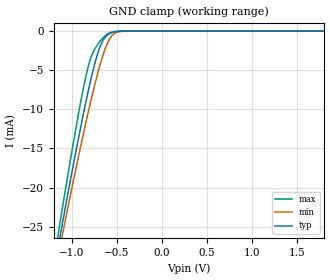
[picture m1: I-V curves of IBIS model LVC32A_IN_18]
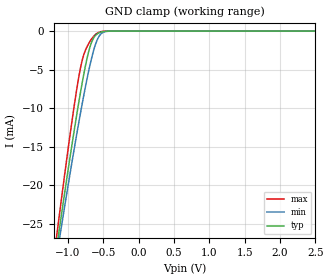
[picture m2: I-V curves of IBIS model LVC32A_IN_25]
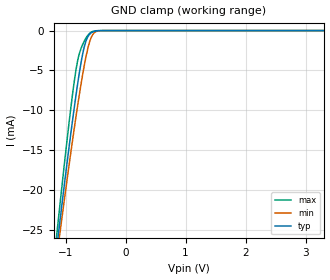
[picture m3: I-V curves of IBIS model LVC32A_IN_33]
| TEXAS INSTRUMENTS INCORPORATED
| Standard Linear and Logic Group
| IBIS Model of SN74LVC32A
| QUADRUPLE 2-INPUT POSITIVE-OR GATES
| This file contains package information for the following:
|  SOIC 14-pin (D) package as [Component] LVC32A_D
|  SOP  14-pin (NS) package as [Component] LVC32A_NS
|  SSOP 14-pin (DB) package as [Component] LVC32A_DB
|  TSSOP 14-pin (PW) package as [Component] LVC32A_PW
|  QFN 14-pin (RGY) package as [Componenet] LVC32A_RGY
| This device can be powered at the following Vccs:
|  1.8 volt Vcc
|  2.5 volt Vcc
|  3.3 volt Vcc
| This file provides unique models under the [Model Selector] for each Vcc.
| For operation at a specific Vcc, select the appropriate model after each
| [Model Selector] keyword.
[IBIS Ver]   3.2
[Comment char]  |_char
[File Name]   sn74lvc32a.ibs
[File Rev]   1.2 | k_die
[Date]   August 19, 2003
[Source]   Data created from TI-SPICE simulations at TI-SLL.
[Notes]   The following is an IBIS list for the LVC32A.
   Please contact sllibis@ti.com with questions and
   comments concerning SLL IBIS models.
   - Power clamp data deleted as there is no power-clamp diode.
[Disclaimer] Property of Texas Instruments Incorporated.  Unauthorized
   reproduction and/or distribution is strictly prohibited.
   This product is protected under copyright law.
   Created  2002, (C) Copyright  2002, Texas Instruments
   Incorporated, All Rights Reserved
   UNLESS THERE IS A SIGNED, WRITTEN AGREEMENT TO THE
   CONTRARY, TEXAS INSTRUMENTS (TI) IS PROVIDING THE IBIS
   MODELS  AND WITHOUT ANY WARRANTY, EXPRESSED OR
   IMPLIED.  TI assumes no liability for:
   1) the accuracy of the IBIS models provided to your
   company;
   2) the proper functioning of these IBIS Models in your
   design or for any resulting applications; or
   3) infringement of patents, copyrights or intellectual
   property rights resulting from your use of these IBIS
   models.
   TI provides IBIS Models as a service to our customers.
   You and your company shall not distribute, sell or give
   these models to anyone else without prior written
   permission from TI.
   TI reserves the right to make changes to our products or
   to discontinue any semiconductor product or service
   without notice, and advises our customers to obtain the
   latest version of relevant information to verify, before
   placing orders, that the information being relied on is
   current.
   Please be aware that your receipt and use of the IBIS
   information provided shall serve as acceptance of these
   terms and conditions.  If you do not accept these terms,
   you should return or destroy the IBIS models and any
   other accompanying information immediately.
| Component LVC32A_D 14-pin SOIC
[Component]   LVC32A_D
[Manufacturer]   Texas Instruments, Inc.
[Package]
|   typ   min   max
R_pkg   3.100e-02   2.800e-02   3.400e-02
L_pkg   3.109e-09   2.462e-09   3.889e-09
C_pkg   4.730e-13   3.630e-13   6.280e-13
[Pin]   signal_name   model_name   R_pin   L_pin   C_pin
1   1A   LVC32A_IN   3.300e-02   3.854e-09   6.220e-13
2   1B   LVC32A_IN   3.200e-02   3.188e-09   4.730e-13
3   1Y   LVC32A_OUT   2.800e-02   2.462e-09   3.770e-13
4   2A   LVC32A_IN   3.100e-02   2.596e-09   3.630e-13
5   2B   LVC32A_IN   2.800e-02   2.521e-09   3.720e-13
6   2Y   LVC32A_OUT   3.400e-02   3.250e-09   4.760e-13
7   GND   GND   3.400e-02   3.889e-09   6.280e-13
8   3Y   LVC32A_OUT   3.400e-02   3.889e-09   6.280e-13
9   3A   LVC32A_IN   3.400e-02   3.250e-09   4.760e-13
10   3B   LVC32A_IN   2.800e-02   2.521e-09   3.720e-13
11   4Y   LVC32A_OUT   3.100e-02   2.596e-09   3.640e-13
12   4A   LVC32A_IN   2.800e-02   2.462e-09   3.770e-13
13   4B   LVC32A_IN   3.200e-02   3.188e-09   4.730e-13
14   VCC   POWER   3.300e-02   3.854e-09   6.220e-13
| Component LVC32A_DB 14-pin SSOP
[Component]   LVC32A_DB
[Manufacturer]   Texas Instruments, Inc.
[Package]
|   typ   min   max
R_pkg   4.400e-02   4.100e-02   4.600e-02
L_pkg   3.551e-09   3.258e-09   3.927e-09
C_pkg   4.020e-13   3.600e-13   4.210e-13
[Pin]   signal_name   model_name   R_pin   L_pin   C_pin
1   1A   LVC32A_IN   4.600e-02   3.927e-09   4.080e-13
2   1B   LVC32A_IN   4.400e-02   3.587e-09   4.210e-13
3   1Y   LVC32A_OUT   4.100e-02   3.289e-09   3.980e-13
4   2A   LVC32A_IN   4.200e-02   3.258e-09   3.600e-13
5   2B   LVC32A_IN   4.100e-02   3.286e-09   4.030e-13
6   2Y   LVC32A_OUT   4.400e-02   3.586e-09   4.210e-13
7   GND   GND   4.600e-02   3.927e-09   4.080e-13
8   3Y   LVC32A_OUT   4.600e-02   3.927e-09   4.080e-13
9   3A   LVC32A_IN   4.400e-02   3.586e-09   4.210e-13
10   3B   LVC32A_IN   4.100e-02   3.286e-09   4.030e-13
11   4Y   LVC32A_OUT   4.300e-02   3.258e-09   3.600e-13
12   4A   LVC32A_IN   4.100e-02   3.289e-09   3.980e-13
13   4B   LVC32A_IN   4.400e-02   3.587e-09   4.210e-13
14   VCC   POWER   4.600e-02   3.927e-09   4.080e-13
| Component LVC126A_NS 14-pin SOP
[Component]   LVC32A_NS
[Manufacturer]  Texas Instruments, Inc.
[Package]
|   typ   min   max
R_pkg   4.500e-02   3.900e-02   5.400e-02
L_pkg   3.796e-09   2.561e-09   4.952e-09
C_pkg   5.280e-13   2.880e-13   7.100e-13
[Pin]   signal_name   model_name   R_pin   L_pin   C_pin
1   1A   LVC32A_IN   4.700e-02   4.867e-09   7.060e-13
2   1B   LVC32A_IN   5.100e-02   4.083e-09   5.920e-13
3   1Y   LVC32A_OUT   4.100e-02   2.915e-09   3.760e-13
4   2A   LVC32A_IN   3.900e-02   2.561e-09   2.880e-13
5   2B   LVC32A_IN   4.100e-02   3.101e-09   4.300e-13
6   2Y   LVC32A_OUT   4.700e-02   4.047e-09   5.890e-13
7   GND   GND   5.100e-02   4.909e-09   7.000e-13
8   3Y   LVC32A_OUT   4.500e-02   4.784e-09   6.940e-13
9   3A   LVC32A_IN   5.400e-02   4.176e-09   5.970e-13
10   3B   LVC32A_IN   3.900e-02   3.287e-09   4.490e-13
11   4Y   LVC32A_OUT   3.900e-02   2.586e-09   2.940e-13
12   4A   LVC32A_IN   4.000e-02   2.802e-09   3.710e-13
13   4B   LVC32A_IN   4.900e-02   4.080e-09   5.930e-13
14   VCC   POWER   5.200e-02   4.952e-09   7.100e-13
| Component LVC32A_PW 14-pin TSSOP
[Component]   LVC32A_PW
[Manufacturer]   Texas Instruments, Inc.
[Package]
|   typ   min   max
R_pkg   3.200e-02   2.900e-02   3.500e-02
L_pkg   2.378e-09   2.170e-09   2.680e-09
C_pkg   3.140e-13   2.700e-13   3.350e-13
[Pin]   signal_name   model_name   R_pin   L_pin   C_pin
1   1A   LVC32A_IN   3.300e-02   2.618e-09   3.300e-13
2   1B   LVC32A_IN   3.100e-02   2.313e-09   3.170e-13
3   1Y   LVC32A_OUT   3.000e-02   2.310e-09   3.140e-13
4   2A   LVC32A_IN   3.100e-02   2.173e-09   2.720e-13
5   2B   LVC32A_IN   3.000e-02   2.204e-09   3.090e-13
6   2Y   LVC32A_OUT   3.200e-02   2.315e-09   3.170e-13
7   GND   GND   3.500e-02   2.680e-09   3.350e-13
8   3Y   LVC32A_OUT   3.300e-02   2.640e-09   3.330e-13
9   3A   LVC32A_IN   3.400e-02   2.347e-09   3.190e-13
10   3B   LVC32A_IN   2.900e-02   2.277e-09   3.130e-13
11   4Y   LVC32A_OUT   3.100e-02   2.170e-09   2.700e-13
12   4A   LVC32A_IN   3.100e-02   2.244e-09   3.110e-13
13   4B   LVC32A_IN   3.300e-02   2.343e-09   3.210e-13
14   VCC   POWER   3.500e-02   2.657e-09   3.320e-13
| Component LVC32A_RGY 14-pin
[Component]   LVC32A_RGY
[Manufacturer]   Texas Instruments, Inc.
[Package]
|   typ   min   max
R_pkg   0.029   0.023   0.041
L_pkg   0.773e-09   0.657e-09   0.998e-09
C_pkg   0.136e-12   0.115e-12   0.156e-12
[Pin]   signal_name   model_name   R_pin   L_pin   C_pin
1   1A   LVC32A_IN   0.027   0.831e-09   0.130e-12
2   1B   LVC32A_IN   0.027   0.866e-09   0.135e-12
3   1Y   LVC32A_OUT   0.041   0.998e-09   0.156e-12
4   2A   LVC32A_IN   0.031   0.767e-09   0.142e-12
5   2B   LVC32A_IN   0.031   0.765e-09   0.142e-12
6   2Y   LVC32A_OUT   0.031   0.783e-09   0.144e-12
7   GND   GND   0.031   0.781e-09   0.137e-12
8   3Y   LVC32A_OUT   0.023   0.657e-09   0.115e-12
9   3A   LVC32A_IN   0.023   0.814e-09   0.129e-12
10   3B   LVC32A_IN   0.028   0.704e-09   0.129e-12
11   4Y   LVC32A_OUT   0.027   0.672e-09   0.136e-12
12   4A   LVC32A_IN   0.027   0.696e-09   0.138e-12
13   4B   LVC32A_IN   0.027   0.725e-09   0.140e-12
14   VCC   POWER   0.030   0.763e-09   0.136e-12
| Model LVC32A_IN
[Model Selector]   LVC32A_IN
LVC32A_IN_18   1.8 volt Vcc
LVC32A_IN_25   2.5 volt Vcc
LVC32A_IN_33   3.3 volt Vcc
| Model LVC32A_OUT
[Model Selector]   LVC32A_OUT
LVC32A_OUT_18   1.8 volt Vcc
LVC32A_OUT_25   2.5 volt Vcc
LVC32A_OUT_33   3.3 volt Vcc
| Models and submodels in the file (6): LVC32A_IN_18 (Input), LVC32A_IN_25 (Input), LVC32A_IN_33 (Input), LVC32A_OUT_18 (Output), LVC32A_OUT_25 (Output), LVC32A_OUT_33 (Output)
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[Model]   LVC32A_IN_18
Model_type  Input
Vinl=0.5775
Vinh=1.2675
| variable   typ   min   max
C_comp   2.66pF   2.19pF   3.17pF
[Temperature Range]   40   100   -40
| Ambient temperature   25   85   -40
[Voltage range]   1.8   1.65   1.95
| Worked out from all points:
|   GND clamp passes 1 mA (typ) near -0.64 V on its own axis
[GND Clamp]
| LVC32A_IN_18
|   Voltage   I(typ)   I(min)   I(max)
-5.5V     -338.9mA   -314.3mA   -369mA
-1.16V    -28.09mA   -29.24mA   -26.56mA
-1.12V    -25.56mA   -26.92mA   -23.71mA
-1.085V   -23.36mA   -24.91mA   -21.25mA
-925mV    -13.65mA   -15.98mA   -10.52mA
-820mV    -7.797mA   -10.48mA   -4.654mA
-770mV    -5.293mA   -8.026mA   -2.891mA
-695mV    -2.253mA   -4.666mA   -1.432mA
-600mV    -473.7uA   -1.449mA   -358.4uA
-535mV    -136.2uA   -379.8uA   -78.5uA
-445mV    -16.2uA    -36.49uA   -4.833uA
1.8V      41.95pA    147.4pA    23.47pA
[Model]   LVC32A_IN_25
Model_type  Input
Vinl=0.7
Vinh=1.7
| variable   typ   min   max
C_comp   2.58pF   2.03pF   3.24pF
[Temperature Range]   40   100   -40
| Ambient temperature   25   85   -40
[Voltage range]   2.5   2.3   2.7
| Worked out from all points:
|   GND clamp passes 1 mA (typ) near -0.64 V on its own axis
[GND Clamp]
| LVC32A_IN_25
|   Voltage   I(typ)   I(min)   I(max)
-5.5V     -338.9mA   -314.3mA   -369mA
-1.17V    -28.73mA   -29.82mA   -27.27mA
-1.13V    -26.19mA   -27.5mA    -24.42mA
-1.095V   -23.98mA   -25.48mA   -21.95mA
-925mV    -13.65mA   -15.98mA   -10.52mA
-825mV    -8.06mA    -10.74mA   -4.88mA
-775mV    -5.531mA   -8.266mA   -3.027mA
-700mV    -2.416mA   -4.874mA   -1.51mA
-590mV    -396.4uA   -1.217mA   -293.2uA
-515mV    -88.16uA   -231.8uA   -44.89uA
-395mV    -4.232uA   -9.445uA   -775nA
2.5V      57.25pA    176.8pA    32.61pA
[Model]   LVC32A_IN_33
Model_type  Input
Vinl=0.8
Vinh=2.0
| variable   typ   min   max
C_comp   2.50pF   1.92pF   3.16pF
[Temperature Range]   40   100   -40
| Ambient temperature   25   85   -40
[Voltage range]   3.3   3   3.6
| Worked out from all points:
|   GND clamp passes 1 mA (typ) near -0.64 V on its own axis
[GND Clamp]
| LVC32A_IN_33
|   Voltage   I(typ)   I(min)   I(max)
-5.5V     -338.9mA   -314.3mA   -369mA
-1.14V    -26.82mA   -28.07mA   -25.13mA
-1.105V   -24.61mA   -26.05mA   -22.65mA
-1.075V   -22.73mA   -24.34mA   -20.55mA
-915mV    -13.07mA   -15.45mA   -9.893mA
-860mV    -9.954mA   -12.53mA   -6.658mA
-805mV    -7.019mA   -9.733mA   -4.027mA
-730mV    -3.528mA   -6.174mA   -2.02mA
-665mV    -1.428mA   -3.486mA   -1.009mA
-585mV    -362.1uA   -1.111mA   -263.9uA
-510mV    -78.77uA   -204.1uA   -38.82uA
3.3V      76.2pA     212.8pA    43.07pA
